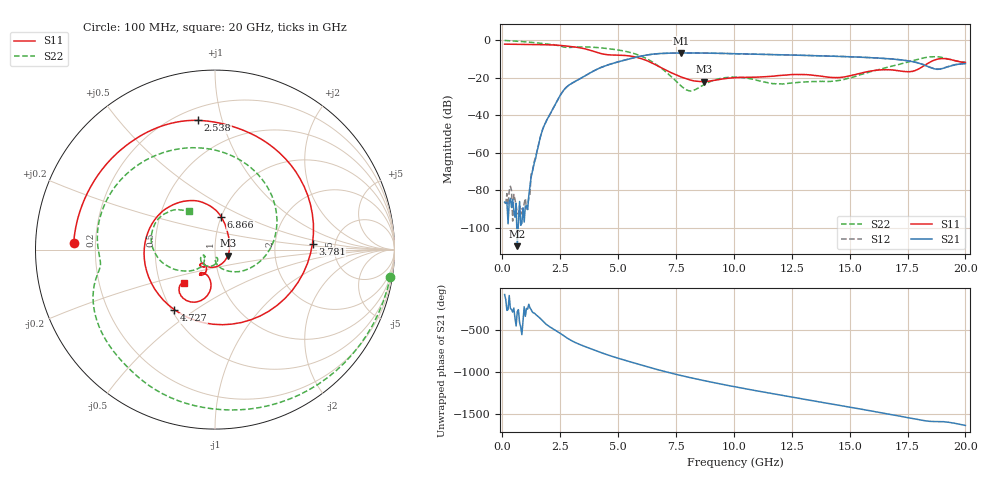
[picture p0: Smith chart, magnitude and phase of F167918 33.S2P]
!  2-Port S-parameters saved by WinCal
! VAR MeasName=S-Parameters (CALIBRATED_DATA) read from VNA (N5242A)
! VAR MeasDate=2016-11-22 10:26:20
! VAR NAME=F167918 33
! VAR FILENAME=F167918 33.S2P
! VAR DATE=2016-11-22 10:26:20
! VAR PHYS_PORTS=1,2
# Hz S DB R 50
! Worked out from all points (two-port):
!   401 points, 100 MHz to 20 GHz, reference 50 ohm
!   highest |S21| = -6.77 dB at 7.712 GHz (marker M1); lowest = -109.9 dB at 647.2 MHz (marker M2)
!   |S21| within 3 dB of the highest: 5.535 GHz to 16.54 GHz (11 GHz wide, 99.7 % of centre)
!   lowest |S11| = -22.1 dB at 8.707 GHz (marker M3), VSWR 1.17, Z = 57.5 - j3.82 ohm
!   |S11| at or under -10 dB: 6.051 GHz to 18.83 GHz (12.78 GHz wide, 103 % of centre); 19.24 GHz to end of sweep
!   |S22| runs from -27.1 to -0.1 dB; largest |S21 - S12| = 0.0049
!   S11 on the Smith chart (normalised r, x): 100 MHz: 0.12, +0.02; 2.538 GHz: 0.28, +0.84; 3.781 GHz: 3.36, +0.31; 4.727 GHz: 0.52, -0.42; 6.866 GHz: 1.00, +0.38; 20 GHz: 0.66, -0.27
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1e8  -2.07 177.3  -86.41 -79.3  -87.19 88.4  -0.10 -8.8
6.4725e8  -2.15 162.7  -109.94 77.6  -92.50 103.8  -0.49 -52.4
1.095e9  -2.22 150.4  -90.41 107.0  -87.85 105.9  -0.94 -84.6
1.74175e9  -2.36 130.4  -47.61 -32.8  -47.62 -33.6  -1.72 -124.6
2.53775e9  -2.78 97.5  -28.68 171.6  -28.69 171.3  -3.26 -165.7
3.43325e9  -4.20 39.6  -19.99 35.7  -20.01 35.8  -3.54 163.8
3.7815e9  -5.28 3.5  -17.49 -1.5  -17.49 -1.2  -3.63 148.2
4.279e9  -7.15 -63.0  -14.46 -52.5  -14.41 -52.3  -4.08 124.9
4.72675e9  -7.87 -124.0  -12.53 -94.8  -12.46 -94.9  -4.70 102.8
5.22425e9  -8.05 -176.7  -10.80 -136.9  -10.75 -137.4  -5.67 75.4
5.82125e9  -9.17 136.1  -8.89 175.0  -8.90 174.5  -7.64 36.4
6.7665e9  -14.01 83.1  -7.10 101.1  -7.15 101.0  -13.97 -35.5
6.866e9  -14.66 79.1  -7.02 93.8  -7.08 93.6  -14.88 -43.0
7.71175e9  -19.54 44.8  -6.77 35.6  -6.80 35.7  -24.27 -88.7
8.70675e9  -22.12 -24.9  -6.83 -24.9  -6.84 -24.9  -23.70 -78.1
1.005e10  -19.94 -100.4  -7.15 -99.2  -7.15 -99.1  -19.66 -129.7
1.1642e10  -19.24 -121.7  -7.63 -179.8  -7.62 -179.8  -23.04 -153.4
1.338325e10  -18.66 -134.9  -8.19 95.7  -8.15 95.9  -22.06 -144.0
1.51245e10  -18.60 -113.6  -8.87 12.6  -8.84 12.4  -19.74 -128.7
1.67165e10  -15.81 -121.4  -9.86 -65.8  -9.89 -65.9  -14.18 -142.0
1.845775e10  -11.76 -99.3  -14.44 -150.6  -14.32 -150.7  -8.86 171.0
2e10  -11.87 -132.5  -12.45 160.1  -12.37 159.8  -11.72 123.8
